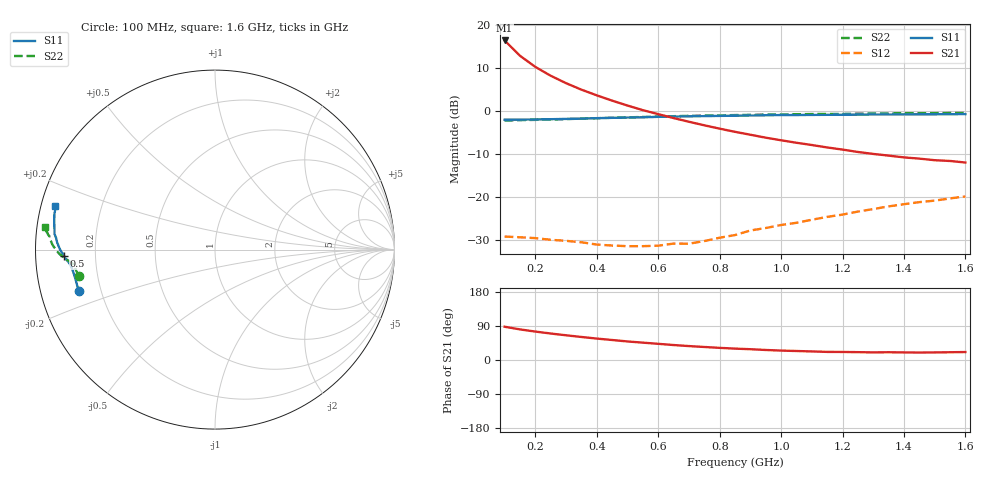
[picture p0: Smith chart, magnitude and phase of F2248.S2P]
! Date: Mon Aug 14 14:20:21 1995
# MHZ  S  MA  R  50.0000
!  POLYFET RF DEVICES
!  F2248
!  S PARAMETERS
!  VDS=12.5V, IDQ=800mA
! FREQ  S11MAG  S11ANG  S21MAG  S21ANG  S12MAG  S12ANG  S22MAG  S22ANG
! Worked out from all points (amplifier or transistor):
!   31 points, 100 MHz to 1.6 GHz, reference 50 ohm
!   highest |S21| = 16.4 dB at 100 MHz (marker M1)
!   |S21| within 3 dB of that: start of sweep to 142.2 MHz
!   unconditionally stable (mu >= 1): 467.6 MHz to 881 MHz
!   at 350 MHz: K = 0.74, MSG = 17.7 dB, |S12| = -30.5 dB
!   at 850 MHz: K = 1.06, MAG = 10.5 dB, |S12| = -28.8 dB
!   at 1.6 GHz: K = 0.58, MSG = 3.9 dB, |S12| = -19.8 dB
!   S11 on the Smith chart (normalised r, x): 100 MHz: 0.12, -0.15; 500 MHz: 0.09, -0.02; 1.6 GHz: 0.04, +0.13
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100  0.7941 -163.0  6.622 87.8  0.03479 7.5  0.7741 -169.0
150  0.7946 -168.3  4.398 80.8  0.03413 5.4  0.7847 -172.1
200  0.7997 -171.1  3.263 75.0  0.03336 4.7  0.7904 -173.6
250  0.8046 -172.6  2.575 69.9  0.0319 6.0  0.7983 -174.4
300  0.8108 -174.0  2.111 65.2  0.03102 8.3  0.8064 -174.9
350  0.8174 -175.0  1.774 60.8  0.02984 9.5  0.8173 -175.5
400  0.8274 -176.0  1.524 56.5  0.0281 13.0  0.8259 -176.0
450  0.8345 -176.5  1.322 52.8  0.02734 17.8  0.836 -176.5
500  0.8412 -177.5  1.16 48.9  0.02689 22.3  0.8461 -177.1
550  0.8466 -178.4  1.025 45.8  0.02689 29.1  0.8542 -177.7
600  0.857 -179.2  0.9212 42.7  0.02723 35.0  0.8627 -178.1
650  0.8626 -179.9  0.8296 39.5  0.0288 39.3  0.8724 -178.8
700  0.8684 179.2  0.7514 36.7  0.02874 44.9  0.8798 -179.4
750  0.8737 178.4  0.6835 34.4  0.03083 50.4  0.8871 179.9
850  0.8838 176.7  0.5738 30.0  0.03621 58.6  0.8989 179.0
900  0.8878 175.8  0.531 28.5  0.04092 60.1  0.9039 178.4
1000  0.8989 174.3  0.4577 24.9  0.04738 64.6  0.9128 177.3
1100  0.9023 172.5  0.4032 22.6  0.05457 67.0  0.9238 176.2
1150  0.9048 171.7  0.3777 21.4  0.05885 67.5  0.9272 175.8
1350  0.9131 168.6  0.3036 20.5  0.07801 68.0  0.9385 174.3
1450  0.9166 167.1  0.2801 19.7  0.08739 67.1  0.9457 173.5
1600  0.922 164.6  0.2523 21.0  0.1018 65.9  0.9533 172.5
